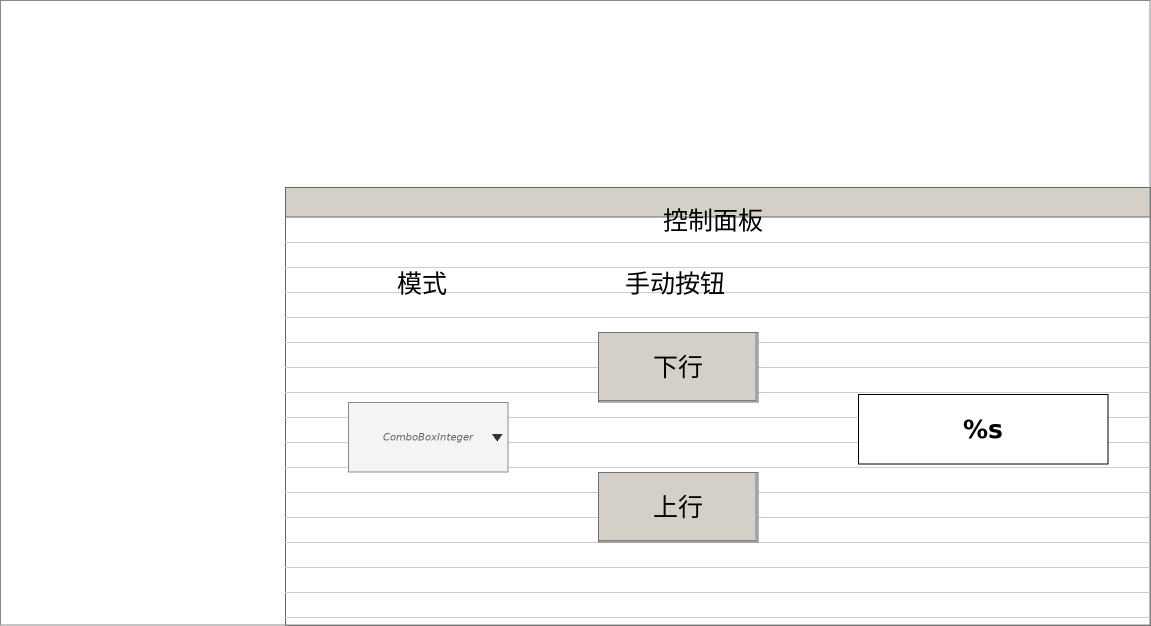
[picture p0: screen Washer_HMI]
VISUALIZATION Washer_HMI  // 1151x626
    Table (285,187 866x439)
    Label (630,201 166x39), "控制面板"
    Button (598,332 160x70), "下行"
        tap Mannual.move_down
    Button (598,472 160x70), "上行"
        tap Mannual.move_up
    Label (600,266 150x35), "手动按钮"
    ComboBoxInteger (348,402 160x70), variable: MAIN.mode_state, text list: 'work_mode'
    Label (347,266 150x35), "模式"
    Rectangle (858,394 250x70), "%s", text variable: Auto.ierrorID, text list: 'Error_ID', text index: Auto.ierrorID
END_VISUALIZATION
